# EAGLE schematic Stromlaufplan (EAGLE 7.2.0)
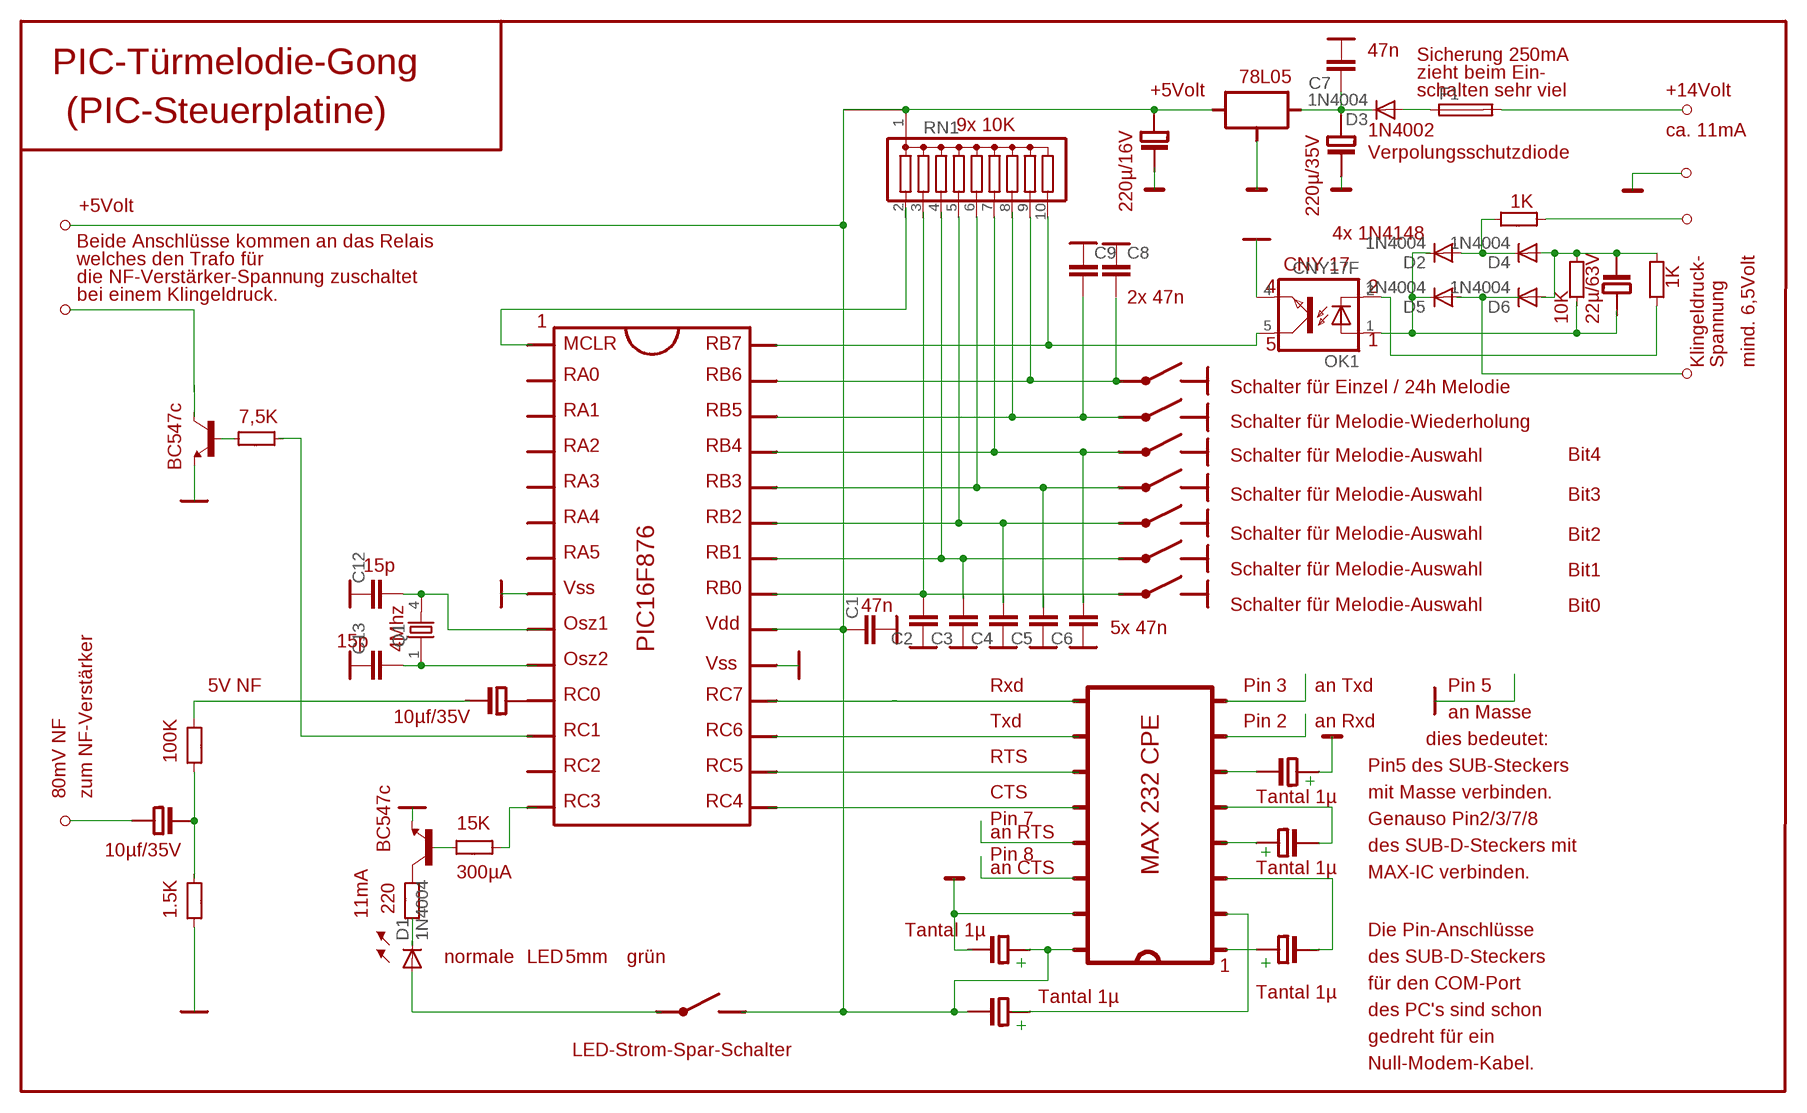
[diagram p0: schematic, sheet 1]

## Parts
C1  C2,5-3  [C2.5-3]
C2  C2,5-3  [C2.5-3]
C3  C2,5-3  [C2.5-3]
C4  C2,5-3  [C2.5-3]
C5  C2,5-3  [C2.5-3]
C6  C2,5-3  [C2.5-3]
C7  C2,5-3  [C2.5-3]
C8  C2,5-3  [C2.5-3]
C9  C2,5-3  [C2.5-3]
C12  C2,5-3  [C2.5-3]
C13  C2,5-3  [C2.5-3]
D1  1N4004  [DO41-10]
D2  1N4004  [DO41-10]
D3  1N4004  [DO41-10]
D4  1N4004  [DO41-10]
D5  1N4004  [DO41-10]
D6  1N4004  [DO41-10]
F1  19559  [19559]
OK1  CNY17F  [DIL06]
Q1  86SMX  [86SMX]
RN1  G09R  [SIL10]

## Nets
N$6: D2.A D4.C
N$9: D1.C
N$12: C2.2 C3.2 C4.2 C5.2 C6.2 RN1.3
N$13: RN1.4
N$18: RN1.5 RN1.6
N$21: RN1.7
N$32: C12.2 Q1.4
N$33: C13.2 Q1.1
N$38: OK1.5(COL)
N$47: D3.A F1.1
N$48: F1.2
N$57: RN1.2
N$58: D5.A D6.C
N$59: D2.C D5.C OK1.1(A)
N$60: C7.1 D3.C
N$61: D4.A D6.A
N$63: OK1.2(C)
N$64: OK1.4(EMIT)
N$65: RN1.8
N$66: D1.A
N$67: C1.1
N$69: C9.2
Unconnected: C1.2 C2.1 C3.1 C4.1 C5.1 C6.1 C7.2 C8.1 C8.2 C9.1 C12.1 C13.1 RN1.1 RN1.9 RN1.10

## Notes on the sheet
- 47n
- Sicherung 250mA
- PIC-Türmelodie-Gong | zieht beim Ein-
- 78L05
- +5Volt | schalten sehr viel | +14Volt
- (PIC-Steuerplatine)
- 9x 10K | 1N4002 | ca. 11mA
- Verpolungsschutzdiode
- 1K
- +5Volt | 220µ/16V | 220µ/35V
- 4x 1N4148
- Beide Anschlüsse kommen an das Relais
- welches den Trafo für | CNY 17
- die NF-Verstärker-Spannung zuschaltet | 1K
- 4 | 2
- bei einem Klingeldruck. | 2x 47n
- 1 | 10K | 22µ/63V
- MCLR | RB7 | 5 | 1
- Klingeldruck- | Spannung | mind. 6,5Volt
- RA0 | RB6
- Schalter für Einzel / 24h Melodie
- BC547c
- RA1 | RB5
- 7,5K | Schalter für Melodie-Wiederholung
- RA2 | RB4
- Schalter für Melodie-Auswahl | Bit4
- RA3 | RB3
- Schalter für Melodie-Auswahl | Bit3
- RA4 | RB2
- Schalter für Melodie-Auswahl | Bit2
- RA5 | RB1
- 15p | Schalter für Melodie-Auswahl | Bit1
- Vss | RB0
- 47n | Schalter für Melodie-Auswahl | Bit0
- Osz1 | Vdd | 5x 47n
- 15p | 4Mhz | PIC16F876
- Osz2 | Vss
- 5V NF | Rxd | Pin 3 | an Txd | Pin 5
- RC0 | RC7
- 10µf/35V | MAX 232 CPE
- an Masse
- Txd | Pin 2 | an Rxd
- RC1 | RC6
- dies bedeutet:
- 100K | RTS
- RC2 | RC5 | Pin5 des SUB-Steckers
- BC547c | Tantal 1µ
- 80mV NF | zum NF-Verstärker | CTS | mit Masse verbinden.
- RC3 | RC4
- 15K | Pin 7 | Genauso Pin2/3/7/8
- 10µf/35V | an RTS
- des SUB-D-Steckers mit
- Pin 8 | Tantal 1µ
- 300µA | an CTS | MAX-IC verbinden.
- 1.5K | 11mA | 220
- Tantal 1µ
- Die Pin-Anschlüsse
- normale | LED | 5mm | grün
- 1 | des SUB-D-Steckers
- Tantal 1µ | Tantal 1µ | für den COM-Port
- des PC's sind schon
- gedreht für ein
- LED-Strom-Spar-Schalter
- Null-Modem-Kabel.

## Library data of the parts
C1-C9 C12 C13 = capacitor-wima:C: CAPACITOR
D1-D6 = diode:1N4004: DIODE
F1 = fuse:19559: FUSE HOLDER
OK1 = optocoupler:CNY17F: SIEMENS OPTO COUPLER
Q1 = crystal:86SMX: CRYSTAL
RN1 = resistor-sil:G09R: SIL RESISTOR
